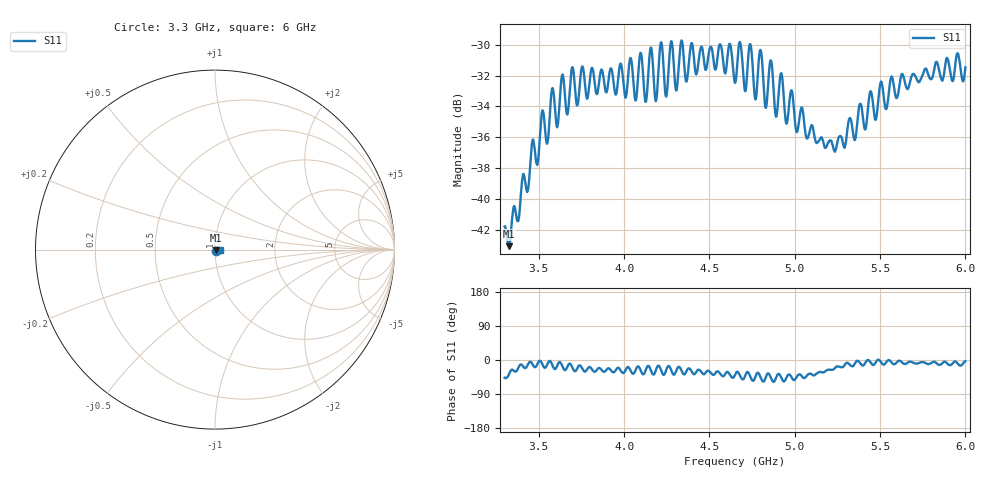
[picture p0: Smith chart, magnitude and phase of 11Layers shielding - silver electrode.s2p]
!  08/07/2025  15:06:46
! Ref Plane: 0.000 mm
# MHZ S MA R  50
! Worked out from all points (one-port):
!   1001 points, 3.3 GHz to 6 GHz, reference 50 ohm
!   lowest |S11| = -43.0 dB at 3.327 GHz (marker M1), VSWR 1.01, Z = 50.6 - j0.415 ohm
!   |S11| at or under -10 dB: start of sweep to end of sweep
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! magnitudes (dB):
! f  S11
! 3.3 GHz  -41.8
! 3.327 GHz  -43.0
! 3.638 GHz  -32.0
! 3.975 GHz  -31.3
! 4.067 GHz  -33.6
! 4.099 GHz  -30.6
! 4.126 GHz  -33.7
! 4.159 GHz  -30.2
! 4.186 GHz  -33.7
! 4.218 GHz  -29.8
! 4.248 GHz  -33.4
! 4.277 GHz  -29.8
! 4.312 GHz  -32.5
! 4.337 GHz  -29.7
! 4.65 GHz  -32.5
! 4.739 GHz  -30.0
! 4.769 GHz  -33.5
! 4.798 GHz  -30.3
! 4.831 GHz  -34.1
! 4.861 GHz  -31.0
! 4.89 GHz  -34.7
! 4.92 GHz  -31.8
! 4.95 GHz  -35.1
! 4.987 GHz  -33.2
! 5.182 GHz  -36.7
! 5.325 GHz  -34.8
! 5.662 GHz  -32.9
! 6 GHz  -31.5
